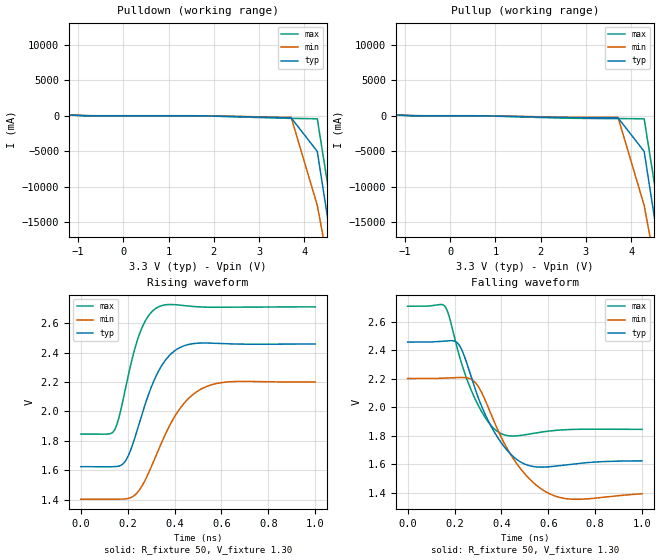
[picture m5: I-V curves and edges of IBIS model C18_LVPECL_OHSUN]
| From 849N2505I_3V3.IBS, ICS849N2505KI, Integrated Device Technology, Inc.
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[Model]   C18_LVPECL_OHSUN
Model_type   Output_ECL
Polarity   Non-Inverting
|   typ   min   max
C_comp   2pF   1.5pF   2.5pF
Vmeas = 2.11V
Rref = 50
Cref = 0
Vref = 1.3V
|   typ   min   max
[Voltage range]   3.3V   3.135V   3.465V
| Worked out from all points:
|   rising waveform, R_fixture 50, V_fixture 1.30: 20-80 % time 113ps typ, 150ps min, 81ps max; typ from 1.62 V to 2.46 V
|   falling waveform, R_fixture 50, V_fixture 1.30: 20-80 % time 127ps typ, 155ps min, 107ps max; typ from 2.46 V to 1.62 V
[Pulldown]
|Voltage   I (typ)   I (min)   I (max)
-3.3V     10.86A     9.972A     12.44A
-2.38V    4.425A     4.618A     4.203A
-1.92V    1.208A     1.942A     478.4mA
-1.46V    201.9mA    181.8mA    231.8mA
-891mV    22.12mA    35.71mA    4.841mA
1.594V    -2.202mA   -809.4uA   -5.593mA
3.71V     -285.4mA   -212.4mA   -370mA
4.288V    -5.015A    -12.6A     -424.4mA
4.866V    -28.68A    -32.33A    -23.64A
6.6V      -99.88A    -91.61A    -114.6A
[Pullup]
|Voltage   I (typ)   I (min)   I (max)
-3.3V     10.86A     9.972A     12.44A
-2.38V    4.425A     4.618A     4.203A
-1.92V    1.208A     1.942A     478.4mA
-1.46V    201.9mA    181.8mA    231.8mA
-891mV    22.12mA    35.71mA    4.841mA
621.3mV   -4.162mA   -1.638mA   -8.972mA
3.71V     -291.7mA   -214.6mA   -397.9mA
4.288V    -5.016A    -12.6A     -425.8mA
4.866V    -28.68A    -32.34A    -23.64A
6.6V      -99.89A    -91.63A    -114.6A
[Ramp]
|   typ   min   max
dV/dt_r   0.673/0.173n   0.641/0.228n   0.705/0.125n
dV/dt_f   0.71/0.203n   0.684/0.25n   0.738/0.168n
R_load =   50.0000
[Rising Waveform]
R_fixture = 50
V_fixture = 1.30   | VCC_typ - 2V
V_fixture_max = 1.465   | VCC_max - 2V
V_fixture_min = 1.135   | VCC_min - 2V
C_fixture = 0.0p
| Time   typ   min   max
0s        1.624V     1.403V     1.846V
143.1ps   1.624V     1.402V     1.871V
163.2ps   1.628V     1.402V     1.96V
194.2ps   1.672V     1.406V     2.18V
248.2ps   1.911V     1.461V     2.516V
285.3ps   2.098V     1.567V     2.642V
328.3ps   2.263V     1.727V     2.708V
424.4ps   2.435V     2.022V     2.722V
529.5ps   2.465V     2.164V     2.709V
1ns       2.458V     2.2V       2.711V
[Falling Waveform]
R_fixture = 50
V_fixture = 1.30   | VCC_typ - 2V
V_fixture_max = 1.465   | VCC_max - 2V
V_fixture_min = 1.135   | VCC_min - 2V
C_fixture = 0.0p
| Time   typ   min   max
0s        2.459V     2.203V     2.711V
156.2ps   2.467V     2.206V     2.715V
176.2ps   2.469V     2.208V     2.645V
214.2ps   2.45V      2.21V      2.399V
295.3ps   2.095V     2.161V     2.034V
395.4ps   1.761V     1.804V     1.819V
492.5ps   1.607V     1.548V     1.806V
617.6ps   1.586V     1.385V     1.837V
727.7ps   1.607V     1.355V     1.847V
1ns       1.625V     1.394V     1.846V
